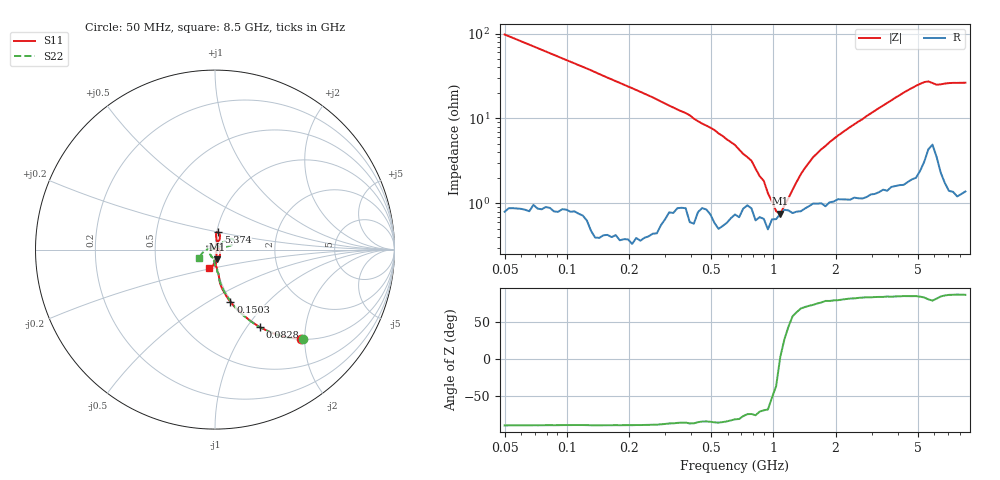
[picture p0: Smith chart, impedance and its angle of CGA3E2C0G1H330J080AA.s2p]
! S-parameter Generated by TDK Corporation
! Copyright(C) 2015 TDK Corporation.
! All Rights Reserved.
! TDK P/N: CGA3E2C0G1H330J080AA (Multilayer Ceramic Chip Capacitors)
! Property: C=33pF
! Size(LxWxT): 1.6x0.8x0.8mm, 0.063x0.031x0.031inches
! Model Type: s2p (Touchstone File Format Version 1.0)
! Frequency: DC=Yes Start=50MHz Stop=8500MHz 114points Log-sweep
! Note:
! Model Generated on Jun. 23, 2015
! Hash(MD5):
! Port Assignments:
!  1 ---| |--- 2
! Applicable Conditions:
!  Temperature = 25 degC
!  DC Bias Voltage = 0 V
!  Small Signal Operation
! Terms and conditions regarding TDK Simulation Models
! (1)This simulation model is being provided solely for informational purposes. Please refer to the specifications of the products in terms of detailed characteristics of such products.
! (2)In no event shall TDK Corporation of any of its subsidiaries be liable for any loss or damage arising, directly or indirectly,
!  From any information contained in this simulation model, including, but not limited to loss or damages arising from any inaccuracies, omissions or errors in connection with such information.
! (3)Any and all copyrights on this simulation model are owned by TDK Corporation.
!  Duplication or redistribution of this simulation model without prior written permission from TDK Corporation is prohibited.
! (4)This simulation model is subject to any modification or change without any prior notice.
! (5)Neither TDK Corporation nor any of its subsidiaries shall make any warranty, express or implied,
!  Including but not limited to the correctness, implied warranties of merchantability and fitness for a particular purpose with respect to this simulation models.
! (6)The use of this simulation model shall be deemed to have consented to the terms and conditions hereof.
# MHz S MA R 50
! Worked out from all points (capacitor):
!   113 points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, 50 MHz to 8.5 GHz, reference 50 ohm
!   read as one part in series: C = 32.6 pF near 50 MHz
!   lowest |Z| = 755 mohm at 1.08 GHz (marker M1)
!   series resonance near 1.076 GHz, so ESL is about 670 pH
!   S11 on the Smith chart (normalised r, x): 50 MHz: 1.01, -1.92; 82.8 MHz: 1.00, -1.15; 150.3 MHz: 0.99, -0.63; 5.374 GHz: 1.02, +0.20; 8.5 GHz: 0.92, -0.20
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50  0.6914 -46.0  0.7106 43.8  0.7112 43.8  0.6984 -45.6
82.80031  0.4992 -60.0  0.8515 29.8  0.8515 29.9  0.51 -59.3
119.495  0.3712 -68.2  0.9145 21.6  0.9136 21.6  0.3826 -67.9
150.2877  0.3032 -73.6  0.9419 17.1  0.9427 17.1  0.3115 -72.5
285.5811  0.1723 -81.7  0.9749 8.1  0.9752 8.1  0.1644 -82.0
651.9202  0.07992 -86.3  0.9825 1.0  0.9819 1.0  0.07528 -92.1
1079.584  0.05474 -79.0  0.9847 -3.0  0.9846 -2.9  0.04674 -106.9
1558.024  0.04545 -63.5  0.9818 -6.0  0.9818 -6.0  0.04032 -124.4
2464.458  0.03481 -36.3  0.9791 -10.8  0.9796 -10.8  0.03173 -151.3
2701.163  0.02985 -25.4  0.9802 -11.9  0.9799 -11.9  0.02623 -159.2
3244.963  0.022 26.6  0.9771 -14.6  0.9773 -14.6  0.01112 115.8
3397.226  0.02624 40.3  0.9772 -15.3  0.9765 -15.4  0.01277 83.7
3723.522  0.03652 66.6  0.9758 -16.9  0.9753 -16.9  0.03157 52.0
4473.143  0.07353 85.4  0.9693 -20.7  0.9713 -20.7  0.07946 39.1
5373.679  0.09794 78.9  0.9517 -25.3  0.952 -25.2  0.1164 30.1
5889.808  0.0607 64.8  0.9347 -26.3  0.9331 -26.2  0.09777 15.0
6455.51  0.0289 79.1  0.9598 -28.1  0.9558 -27.9  0.04324 24.0
6758.422  0.01203 60.8  0.9639 -29.7  0.9649 -29.7  0.02307 44.7
7075.547  0.01354 -50.9  0.9669 -31.3  0.9661 -31.2  0.01614 120.1
7407.553  0.03847 -77.3  0.9667 -33.0  0.9648 -33.0  0.03311 169.2
7755.137  0.06547 -90.3  0.9639 -34.9  0.9637 -34.6  0.0583 -173.5
8500  0.1098 -106.5  0.9604 -38.6  0.9622 -38.5  0.1011 -150.8
